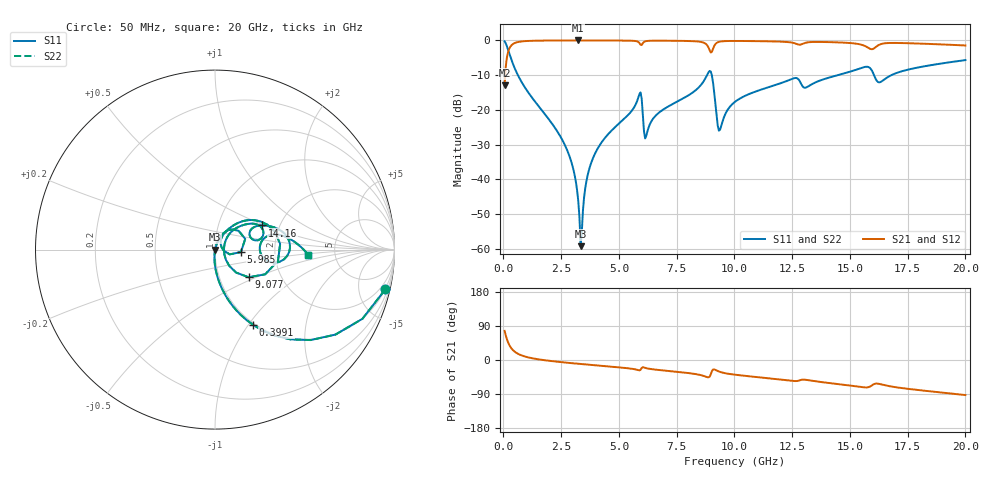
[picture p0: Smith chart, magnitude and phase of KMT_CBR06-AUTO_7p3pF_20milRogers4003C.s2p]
! Data measured by Modelithics Inc. support@modelithics.com 813-866-6335
! KEMET CBR06-AUTO 7.3pF, Pad Width= 0.851mm, Pad Length= 0.64mm, Pad Gap= 0.62mm, 20mil Rogers 4003C substrate Data, January 2022
# hz S ma R 50
! 2 Port Network Data from SP1.SP block
! freq  magS11  angS11  magS21  angS21  magS12  angS12  magS22  angS22
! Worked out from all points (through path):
!   401 points, 50 MHz to 20 GHz, reference 50 ohm
!   highest |S21| = -0.01 dB at 3.242 GHz (marker M1); lowest = -12.9 dB at 50 MHz (marker M2)
!   group delay of S21, straight-line fit = 14.2 ps
!   lowest |S11| = -59.2 dB at 3.342 GHz (marker M3), VSWR 1.00, Z = 50.1 - j0.0737 ohm
!   |S11| at or under -10 dB: 627 MHz to 8.813 GHz (8.186 GHz wide, 173 % of centre); 9.022 GHz to 14.47 GHz (5.446 GHz wide, 46.4 % of centre); 16.04 GHz to 16.79 GHz (747.3 MHz wide, 4.55 % of centre)
!   |S22| runs from -59.2 to -0.2 dB; largest |S21 - S12| = 0
!   S11 on the Smith chart (normalised r, x): 50 MHz: 0.98, -8.54; 399.1 MHz: 0.98, -1.06; 5.985 GHz: 1.34, -0.04; 9.077 GHz: 1.37, -0.45; 14.16 GHz: 1.63, +0.48; 20 GHz: 3.15, -0.26
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5e7  0.9742 -13.2  0.2254 76.8  0.2254 76.8  0.9742 -13.2
3.99125e8  0.4711 -63.1  0.8815 26.8  0.8815 26.8  0.4711 -63.1
2.693375e9  0.02959 -95.2  0.9986 -6.8  0.9986 -6.8  0.02959 -95.2
3.0425e9  0.01328 -95.0  0.9989 -8.8  0.9989 -8.8  0.01328 -95.0
3.242e9  0.004783 -88.9  0.999 -10.0  0.999 -10.0  0.004783 -88.9
3.34175e9  0.001099 -42.0  0.9989 -10.5  0.9989 -10.5  0.001099 -42.0
3.391625e9  0.001731 46.2  0.9989 -10.8  0.9989 -10.8  0.001731 46.2
3.641e9  0.01134 72.9  0.9988 -12.1  0.9988 -12.1  0.01134 72.9
4.04e9  0.02641 73.4  0.9984 -14.3  0.9984 -14.3  0.02641 73.4
5.8355e9  0.1492 48.8  0.9519 -26.7  0.9519 -26.7  0.1492 48.8
5.985125e9  0.1453 -5.4  0.8592 -21.1  0.8592 -21.1  0.1453 -5.4
6.184625e9  0.04258 40.6  0.9792 -21.6  0.9792 -21.6  0.04258 40.6
6.73325e9  0.09147 61.2  0.9917 -26.4  0.9917 -26.4  0.09147 61.2
8.678375e9  0.2619 39.1  0.9256 -42.2  0.9256 -42.2  0.2619 39.1
9.077375e9  0.2423 -39.5  0.7633 -24.9  0.7633 -24.9  0.2423 -39.5
9.376625e9  0.05191 13.2  0.962 -31.4  0.962 -31.4  0.05191 13.2
1.0025e10  0.1309 47.5  0.9827 -38.8  0.9827 -38.8  0.1309 47.5
1.336662e10  0.2361 29.6  0.9495 -55.0  0.9495 -55.0  0.2361 29.6
1.416462e10  0.2963 27.0  0.9448 -61.1  0.9448 -61.1  0.2963 27.0
1.601e10  0.3365 -12.6  0.7569 -64.7  0.7569 -64.7  0.3365 -12.6
1.670825e10  0.3059 14.6  0.9186 -69.1  0.9186 -69.1  0.3059 14.6
2e10  0.5213 -3.3  0.8457 -92.5  0.8457 -92.5  0.5213 -3.3
